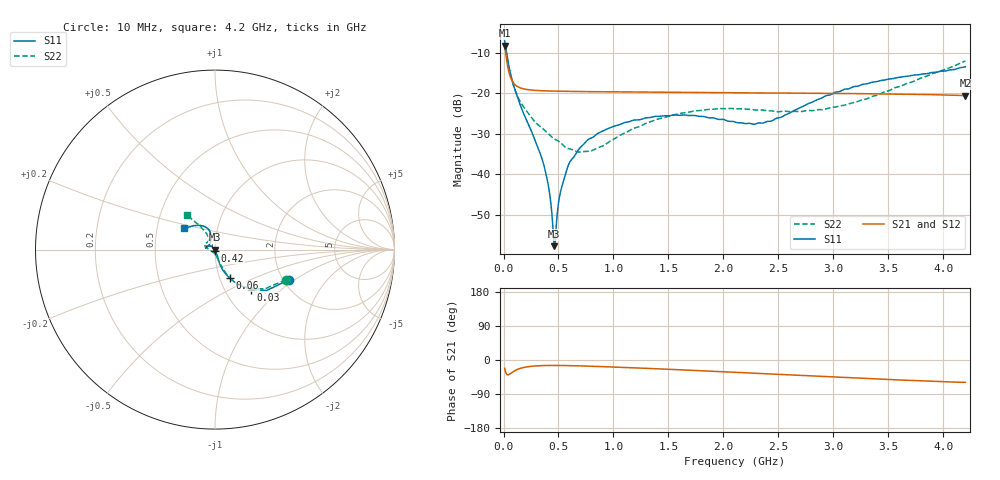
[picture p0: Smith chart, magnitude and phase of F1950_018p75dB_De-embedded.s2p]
! Integrated Device Technology
! Corporate Headquarters
! 6024 Silver Creek Valley Road
! San Jose, CA 95138  USA
! Phone:  1-408-284-8200
! Toll Free:  1-800-223-1366
! Webpage:  http://www.idt.com/
! Timing and RF Division
! 515 Groton Road, Suite 102
! Westford, MA 01886-6024
! Device:  F1950
! Description: 7-bit 0.25 dB Digital Step Attenuator
! Frequency:  150.0 -  4000.00 MHz
! Package:  4x4 mm Thin QFN Plastic Package: 24 pin
! Ports:  2 RF, 12 DC
!  Pin  1  = D0
!  Pin  2  = VDD
!  Pin  3  = Vmode
!  Pin  4  = GND
!  Pin  5  = RF1  =  Port 1
!  Pin  6  = GND
!  Pin  7  = GND
!  Pin  8  = GND
!  Pin  9  = GND
!  Pin 10  = GND
!  Pin 11  = GND
!  Pin 12  = GND
!  Pin 13  = GND
!  Pin 14  = RF2  =  Port 2
!  Pin 15  = GND
!  Pin 16  = LE
!  Pin 17  = CLK
!  Pin 18  = DATE
!  Pin 19  = D6
!  Pin 20  = D5
!  Pin 21  = D4
!  Pin 22  = D3
!  Pin 23  = D2
!  Pin 24  = D1
! State:  75
! Atten State:  18.75 dB
! Voltage:  +5.00 Volts
! Current:  Not Measured mA
! Data:  The device was measured on a the F195X evaluation board which has
!  individual transmission lines to the RF pins.  Data was collected
!  using a calibrated network analyzer.  The evaluation board was
!  de-embedded using a TRL calibration technique.
!  The reference plane is the edge of the package pin.
! Misc:  Board 2019
!  Action Tracker AT0250
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# GHz S dB R 50
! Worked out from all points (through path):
!   420 points, 10 MHz to 4.2 GHz, reference 50 ohm
!   highest |S21| = -8.28 dB at 10 MHz (marker M1); lowest = -20.6 dB at 4.2 GHz (marker M2)
!   group delay of S21, straight-line fit = 30.9 ps
!   lowest |S11| = -57.7 dB at 460 MHz (marker M3), VSWR 1.00, Z = 49.9 - j0.1 ohm
!   |S11| at or under -10 dB: 27.2 MHz to end of sweep
!   |S22| runs from -34.5 to -7.4 dB; largest |S21 - S12| = 0.00018
!   S11 on the Smith chart (normalised r, x): 10 MHz: 2.14, -0.90; 30 MHz: 1.32, -0.64; 60 MHz: 1.12, -0.37; 420 MHz: 1.00, -0.01; 4.2 GHz: 0.68, +0.17
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0.01  -7.03 -22.2  -8.28 -21.8  -8.28 -21.8  -7.35 -23.1
0.03  -10.50 -48.2  -12.09 -38.3  -12.09 -38.3  -10.73 -48.2
0.06  -14.92 -62.6  -15.82 -36.7  -15.82 -36.6  -14.87 -62.0
0.11  -19.61 -70.4  -18.06 -27.1  -18.06 -27.1  -19.63 -68.0
0.17  -24.18 -71.3  -18.87 -20.6  -18.87 -20.7  -22.90 -72.3
0.35  -36.18 -68.4  -19.42 -14.8  -19.42 -14.8  -28.57 -79.1
0.39  -40.44 -69.3  -19.46 -14.5  -19.46 -14.5  -29.55 -80.0
0.42  -44.89 -76.2  -19.49 -14.4  -19.49 -14.4  -30.33 -81.6
0.45  -53.31 -96.6  -19.51 -14.3  -19.51 -14.3  -31.04 -85.4
0.46  -57.72 -129.5  -19.51 -14.3  -19.51 -14.3  -31.23 -86.8
0.48  -52.56 152.2  -19.53 -14.3  -19.53 -14.4  -31.53 -89.3
0.5  -47.07 140.4  -19.54 -14.4  -19.54 -14.4  -31.84 -90.9
0.52  -44.13 138.7  -19.55 -14.4  -19.55 -14.5  -32.24 -91.9
0.57  -39.38 133.9  -19.57 -14.7  -19.57 -14.7  -33.50 -99.6
0.71  -33.10 137.4  -19.62 -15.7  -19.62 -15.7  -34.45 -124.6
0.99  -28.33 147.2  -19.71 -18.5  -19.71 -18.5  -31.54 -169.0
1.41  -25.72 163.2  -19.80 -23.4  -19.80 -23.4  -26.36 167.8
2.11  -27.18 158.5  -19.92 -32.6  -19.92 -32.6  -23.87 149.6
2.43  -26.93 126.4  -19.97 -36.8  -19.97 -36.8  -24.37 140.0
2.81  -22.18 105.2  -20.04 -42.1  -20.04 -42.1  -24.32 125.4
3.51  -16.52 117.5  -20.21 -51.5  -20.21 -51.6  -19.36 118.8
4.2  -13.51 146.1  -20.61 -59.0  -20.61 -59.1  -12.09 129.1
